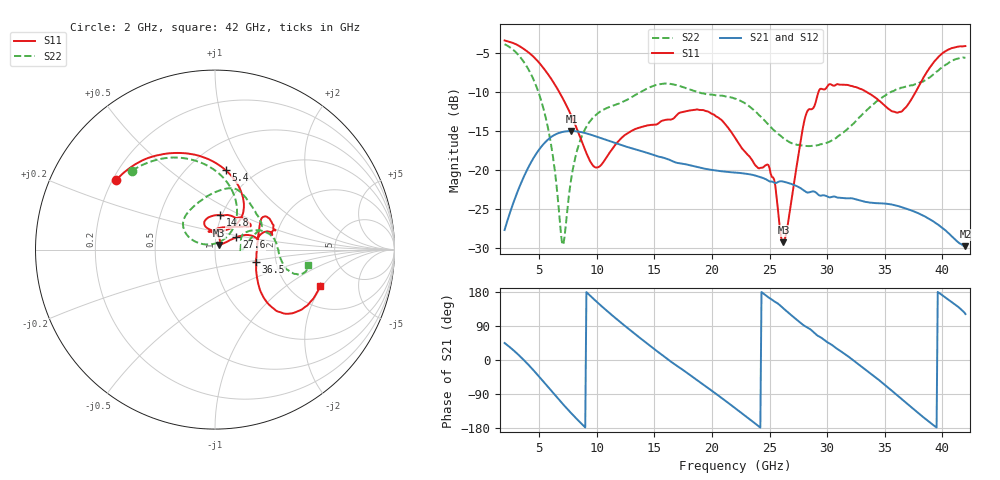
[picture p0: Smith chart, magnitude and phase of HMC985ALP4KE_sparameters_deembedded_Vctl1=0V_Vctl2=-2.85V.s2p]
!s2p File: Measurements: S11, S21, S12, S22
# GHz S dB R 50.0
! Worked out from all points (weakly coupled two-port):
!   401 points, 2 GHz to 42 GHz, reference 50 ohm
!   highest |S21| = -15.04 dB at 7.8 GHz (marker M1); lowest = -29.8 dB at 42 GHz (marker M2)
!   lowest |S11| = -29.3 dB at 26.2 GHz (marker M3), VSWR 1.07, Z = 52.3 + j2.69 ohm
!   |S11| at or under -10 dB: 6.727 GHz to 29.26 GHz (22.53 GHz wide, 125 % of centre); 33.39 GHz to 37.7 GHz (4.309 GHz wide, 12.1 % of centre)
!   |S22| runs from -29.6 to -3.9 dB; largest |S21 - S12| = 0.00068
!   S11 on the Smith chart (normalised r, x): 2 GHz: 0.21, +0.30; 5.4 GHz: 0.74, +0.82; 14.8 GHz: 0.98, +0.39; 27.6 GHz: 1.26, +0.18; 36.5 GHz: 1.57, -0.22; 42 GHz: 2.92, -1.90
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2  -3.43 144.8  -27.72 44.8  -27.70 44.8  -3.91 136.5
3.5  -4.36 118.6  -21.46 5.0  -21.48 5.0  -5.84 103.0
5.4  -7.02 82.2  -16.67 -58.1  -16.70 -58.1  -12.33 59.5
6.2  -8.70 67.9  -15.65 -86.5  -15.63 -86.5  -18.34 47.3
7  -10.72 56.3  -15.16 -114.3  -15.18 -114.4  -29.52 91.1
7.8  -13.11 50.1  -15.04 -140.9  -15.04 -140.9  -20.98 157.5
8.7  -16.37 53.0  -15.19 -169.0  -15.20 -169.0  -15.71 154.2
10.1  -19.69 89.4  -15.81 150.7  -15.78 150.7  -12.75 140.7
14.8  -14.25 81.8  -18.03 33.3  -18.02 33.3  -9.32 81.1
15.4  -14.00 74.0  -18.33 19.6  -18.36 19.5  -9.05 75.9
19.3  -12.38 33.7  -19.84 -65.9  -19.86 -65.9  -10.22 43.2
22  -15.89 52.1  -20.36 -126.7  -20.37 -126.8  -10.89 25.4
25  -19.82 99.3  -21.49 163.4  -21.48 163.4  -14.38 13.7
26.2  -29.27 48.3  -21.52 136.2  -21.53 136.2  -15.95 2.4
27.6  -17.25 30.0  -22.28 100.1  -22.31 100.1  -16.82 -5.0
28.7  -12.22 13.0  -22.78 76.9  -22.76 77.0  -16.92 0.1
31  -9.06 23.2  -23.57 26.9  -23.55 26.9  -15.65 26.0
33.3  -9.92 34.2  -24.11 -24.7  -24.10 -24.7  -12.59 26.9
35.4  -12.27 11.9  -24.41 -75.6  -24.41 -75.6  -10.17 16.9
36.5  -12.51 -16.4  -24.80 -103.9  -24.80 -103.9  -9.46 10.0
39.5  -5.83 -43.4  -26.91 -178.1  -26.87 -178.1  -7.43 -15.7
42  -4.15 -18.8  -29.79 121.3  -29.80 121.2  -5.61 -9.3
